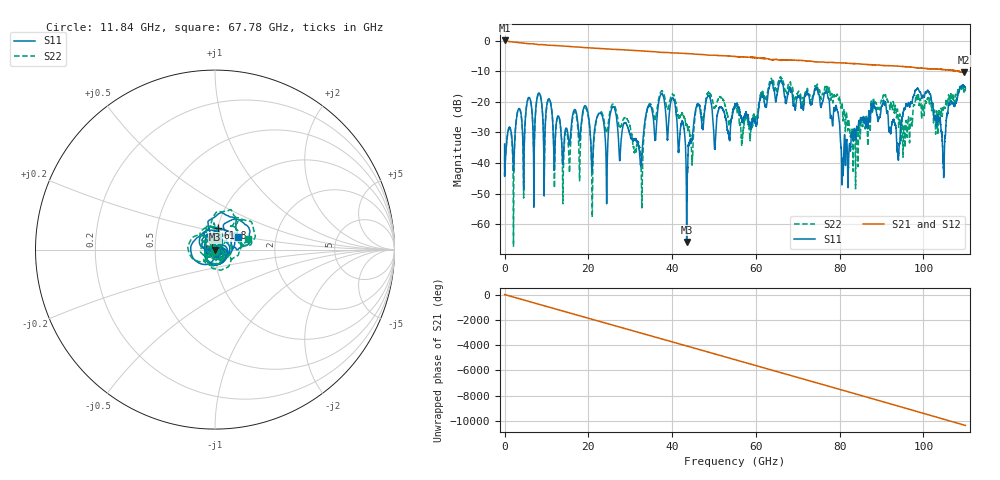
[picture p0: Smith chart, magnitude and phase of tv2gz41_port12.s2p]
!Keysight Technologies,N5247A,US51370218,A.10.49.08
!Posted to IEEE NEA 05/29  by John Calvin
!Date: Wednesday, February 21, 2018 16:45:26
!Correction: S11(Full 2 Port(1,2))
!S21(Full 2 Port(1,2))
!S12(Full 2 Port(1,2))
!S22(Full 2 Port(1,2))
!S2P File: Measurements: S11, S21, S12, S22:
# Hz S  dB  R 50
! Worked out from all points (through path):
!   11000 points, 10 MHz to 110 GHz, reference 50 ohm
!   highest |S21| = 0.06 dB at 10 MHz (marker M1); lowest = -10.4 dB at 109.6 GHz (marker M2)
!   group delay of S21, straight-line fit = 261 ps
!   lowest |S11| = -65.9 dB at 43.47 GHz (marker M3), VSWR 1.00, Z = 50 + j0.0453 ohm
!   |S11| at or under -10 dB: start of sweep to end of sweep
!   |S22| runs from -67.2 to -11.8 dB; largest |S21 - S12| = 0.034
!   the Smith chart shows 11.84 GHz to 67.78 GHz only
!   S11 on the Smith chart (normalised r, x): 11.84 GHz: 1.01, -0.01; 61.8 GHz: 1.01, +0.24; 67.78 GHz: 1.28, +0.18
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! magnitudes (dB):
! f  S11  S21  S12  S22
! 10 MHz  -33.8  0.1  0.0  -37.7
! 8.2 GHz  -17.1  -1.3  -1.3  -17.3
! 11.84 GHz  -42.1  -1.6  -1.6  -42.6
! 18.35 GHz  -26.4  -2.2  -2.2  -27.7
! 24.36 GHz  -53.2  -2.7  -2.7  -30.2
! 25.99 GHz  -21.7  -2.8  -2.8  -20.8
! 32.61 GHz  -40.1  -3.3  -3.4  -42.2
! 36.68 GHz  -21.2  -3.7  -3.7  -19.7
! 40.29 GHz  -19.1  -4.0  -4.0  -17.8
! 43.47 GHz  -65.9  -4.2  -4.2  -27.5
! 46.03 GHz  -20.8  -4.5  -4.5  -21.1
! 55.01 GHz  -20.8  -5.2  -5.2  -22.1
! 61.8 GHz  -18.4  -5.8  -5.8  -17.7
! 67.78 GHz  -16.8  -6.3  -6.3  -14.4
! 73.34 GHz  -20.6  -6.8  -6.8  -19.7
! 79.17 GHz  -21.4  -7.2  -7.2  -18.1
! 80.91 GHz  -39.8  -7.3  -7.3  -23.8
! 91.67 GHz  -28.4  -8.2  -8.2  -20.3
! 101 GHz  -16.2  -9.2  -9.2  -18.7
! 104.8 GHz  -41.3  -9.5  -9.4  -21.9
! 109.6 GHz  -14.8  -10.4  -10.3  -16.4
! 110 GHz  -15.5  -10.3  -10.3  -16.5
